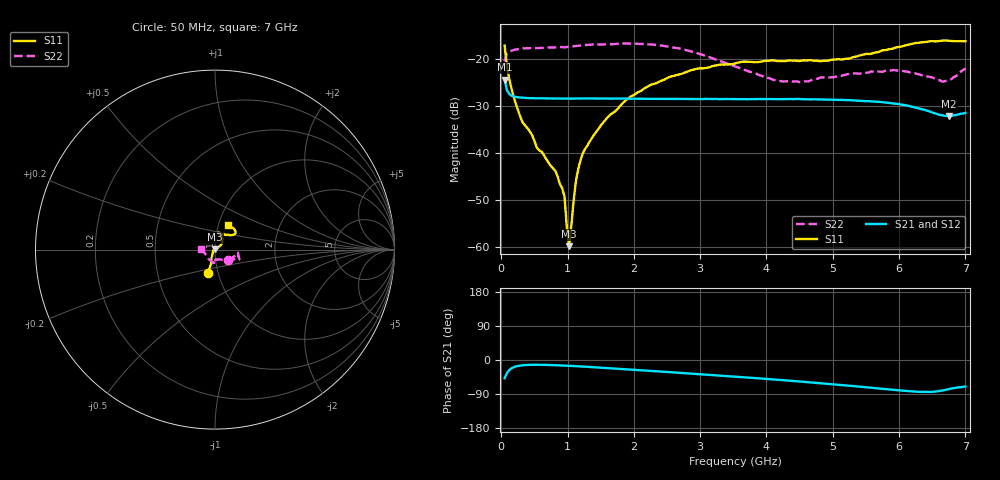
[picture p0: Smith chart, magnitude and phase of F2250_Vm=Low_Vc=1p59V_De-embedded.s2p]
! Integrated Device Technology
! Corporate Headquarters
! 6024 Silver Creek Valley Road
! San Jose, CA 95138  USA
! Phone:  1-408-284-8200
! Toll Free:  1-800-223-1366
! Webpage:  http://www.idt.com/
! Timing and RF Division
! 515 Groton Road, Suite 102
! Westford, MA 01886-6024
! Device:  F2250
! Description: Voltage Variable RF Attenuator
! Frequency:  50.0 -  6000.00 MHz
! Package:  3x3 mm Thin QFN Plastic Package: 16 pin
! Ports:  2 RF, 3 DC
!  Pin  1  = GND
!  Pin  2  = NC
!  Pin  3  = RF1  = Port 1
!  Pin  4  = NC
!  Pin  5  = GND
!  Pin  6  = GND
!  Pin  7  = GND
!  Pin  8  = GND
!  Pin  9  = NC
!  Pin 10  = RF2  = Port 2
!  Pin 11  = NC
!  Pin 12  = GND
!  Pin 13  = GND
!  Pin 14  = VCNTRL
!  Pin 15  = VDD
!  Pin 16  = VMODE
! Vcntrl:  1.590 Volts
! Vmode:  +0.000 Volts
! Vdd:  +3.30  Volts
! Current:  1.189 mA
! Data:  The device was measured on a the F2250 evaluation board which has
!  individual transmission lines to the RF pins.  Data was collected
!  using a calibrated network analyzer.  The evaluation board was
!  de-embedded using a TRL calibration technique.
!  The reference plane is the edge of the package pin.
! Misc:  SN 10
!  Action Tracker AT0258
! Date Measured:  2014-11-26
! Date:  2015-10-15  MJV
! Note:
!  Integrated Device Technology supplies this data as a sample of measured
!  data at the package pin for this product.  Your particular data for this
!  product may vary.
!  Data was taken at 25 degrees C.
!  Integrated Device Technology reserves the right to change this data at anytime.
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# GHz S dB R 50
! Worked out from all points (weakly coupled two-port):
!   201 points, 50 MHz to 7 GHz, reference 50 ohm
!   highest |S21| = -24.39 dB at 50 MHz (marker M1); lowest = -32.2 dB at 6.757 GHz (marker M2)
!   lowest |S11| = -59.9 dB at 1.023 GHz (marker M3), VSWR 1.00, Z = 50 + j0.0988 ohm
!   |S11| at or under -10 dB: start of sweep to end of sweep
!   |S22| runs from -24.9 to -16.7 dB; largest |S21 - S12| = 0.0003
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0.05  -17.17 -107.2  -24.39 -48.1  -24.37 -48.1  -20.52 -39.9
0.1195  -24.26 -109.4  -27.46 -26.5  -27.47 -26.5  -18.44 -11.9
0.29325  -32.60 -122.3  -28.24 -14.5  -28.22 -14.5  -17.77 -8.5
0.467  -36.32 -140.9  -28.36 -12.6  -28.36 -12.6  -17.71 -8.2
0.5365  -38.92 -148.0  -28.40 -12.6  -28.38 -12.6  -17.70 -9.3
0.8145  -43.83 175.9  -28.45 -13.8  -28.44 -13.8  -17.54 -13.3
0.91875  -47.58 155.4  -28.45 -14.5  -28.45 -14.5  -17.47 -15.0
0.9535  -49.32 176.3  -28.47 -14.7  -28.45 -14.8  -17.54 -15.2
0.98825  -55.85 159.4  -28.45 -15.0  -28.44 -15.0  -17.46 -15.5
1.023  -59.90 102.3  -28.45 -15.3  -28.46 -15.3  -17.40 -15.5
1.12725  -45.85 37.1  -28.42 -16.2  -28.42 -16.2  -17.24 -16.9
1.2315  -40.04 31.4  -28.43 -17.2  -28.44 -17.3  -17.08 -18.4
1.61375  -32.27 35.5  -28.45 -21.4  -28.47 -21.4  -16.90 -20.7
1.9265  -28.25 37.9  -28.49 -25.0  -28.50 -25.0  -16.72 -22.1
2.37825  -24.87 45.0  -28.49 -30.2  -28.51 -30.2  -17.07 -23.8
2.93425  -22.13 58.3  -28.55 -36.7  -28.55 -36.7  -18.68 -27.3
3.525  -20.96 71.4  -28.56 -44.0  -28.58 -43.9  -21.60 -42.1
4.11575  -20.32 79.0  -28.58 -51.4  -28.58 -51.5  -24.51 -66.0
4.7065  -20.36 71.7  -28.60 -59.8  -28.58 -59.8  -24.37 -91.1
5.85325  -17.92 39.8  -29.39 -77.7  -29.39 -77.7  -22.49 -97.0
6.75675  -16.14 50.7  -32.17 -76.7  -32.18 -76.7  -24.48 -157.3
7  -16.24 62.8  -31.50 -69.9  -31.57 -69.7  -22.05 176.5
